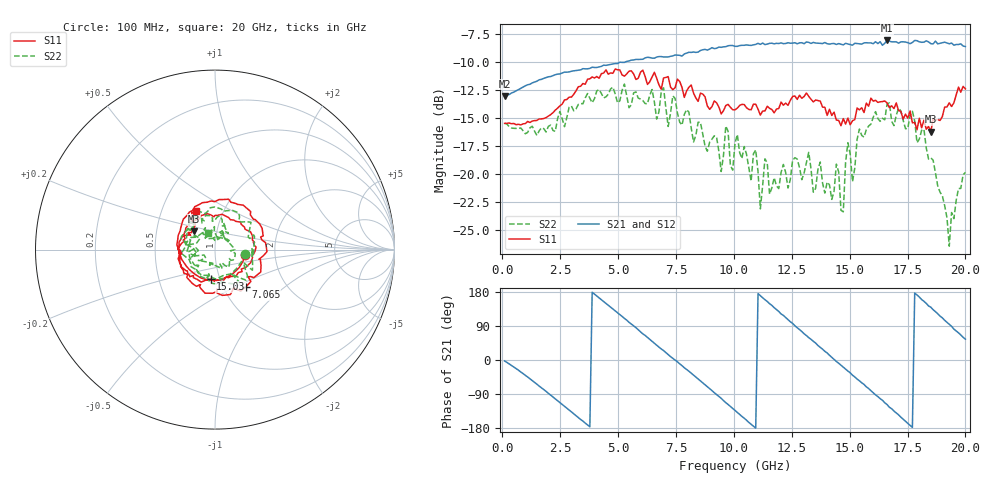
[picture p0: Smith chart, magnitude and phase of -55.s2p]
!Agilent Technologies,N5230C,MY49001569,A.09.33.09
!Agilent N5230C: A.09.33.09
!Date: Monday, July 20, 2015 19:15:45
!Correction: S11(Full 2 Port(1,2))
!S21(Full 2 Port(1,2))
!S12(Full 2 Port(1,2))
!S22(Full 2 Port(1,2))
!S2P File: Measurements: S11, S21, S12, S22:
# Hz S  dB  R 50
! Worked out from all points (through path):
!   201 points, 100 MHz to 20 GHz, reference 50 ohm
!   highest |S21| = -8.10 dB at 16.62 GHz (marker M1); lowest = -13.1 dB at 100 MHz (marker M2)
!   group delay of S21, straight-line fit = 143 ps
!   lowest |S11| = -16.2 dB at 18.51 GHz (marker M3), VSWR 1.37, Z = 38.8 + j8.02 ohm
!   |S11| at or under -10 dB: start of sweep to end of sweep
!   |S22| runs from -26.4 to -12.0 dB; largest |S21 - S12| = 0.015
!   S11 on the Smith chart (normalised r, x): 100 MHz: 1.40, -0.08; 7.065 GHz: 1.27, -0.57; 15.03 GHz: 0.90, -0.30; 20 GHz: 0.74, +0.34
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1e8  -15.49 -9.4  -13.06 -2.5  -13.07 -2.4  -15.47 -7.7
1.5925e9  -15.09 -115.0  -11.61 -68.8  -11.62 -69.0  -16.15 -112.8
3.483e9  -11.94 124.5  -10.61 -161.2  -10.69 -161.5  -13.74 129.3
5.3735e9  -11.08 36.9  -9.97 105.2  -10.04 104.8  -13.04 30.1
6.7665e9  -12.06 -37.0  -9.54 34.1  -9.52 34.0  -14.45 -30.1
7.065e9  -11.39 -50.4  -9.57 19.5  -9.54 19.4  -14.12 -50.6
8.7565e9  -13.12 -135.3  -8.90 -65.0  -8.91 -65.7  -17.53 -139.8
1.005e10  -14.28 153.0  -8.62 -133.0  -8.62 -133.4  -17.27 144.7
1.07465e10  -14.27 115.6  -8.54 -169.8  -8.53 -169.8  -20.63 113.1
1.09455e10  -13.79 102.1  -8.45 -179.6  -8.42 179.6  -17.85 91.4
1.11445e10  -14.75 92.0  -8.45 169.7  -8.53 168.9  -23.11 80.6
1.1443e10  -13.96 78.7  -8.42 154.4  -8.40 153.6  -19.02 69.2
1.3234e10  -13.08 -3.3  -8.27 58.9  -8.41 59.3  -18.07 -51.7
1.3433e10  -13.57 -9.9  -8.28 49.4  -8.37 48.5  -21.62 -62.1
1.4428e10  -15.19 -59.6  -8.46 -3.8  -8.49 -3.3  -19.12 -147.1
1.47265e10  -15.06 -73.8  -8.50 -19.2  -8.39 -19.1  -23.37 -153.6
1.5025e10  -15.61 -98.6  -8.47 -33.8  -8.28 -34.3  -18.21 -165.2
1.6617e10  -13.66 -167.2  -8.10 -117.5  -8.18 -117.4  -13.77 131.3
1.67165e10  -14.09 -175.1  -8.16 -124.6  -8.17 -124.0  -13.67 117.8
1.85075e10  -16.21 139.3  -8.39 139.3  -8.22 137.8  -18.56 52.1
1.93035e10  -13.66 127.2  -8.40 94.1  -8.32 92.8  -26.43 88.0
2e10  -12.42 115.8  -8.64 54.9  -8.51 53.5  -19.85 113.1
